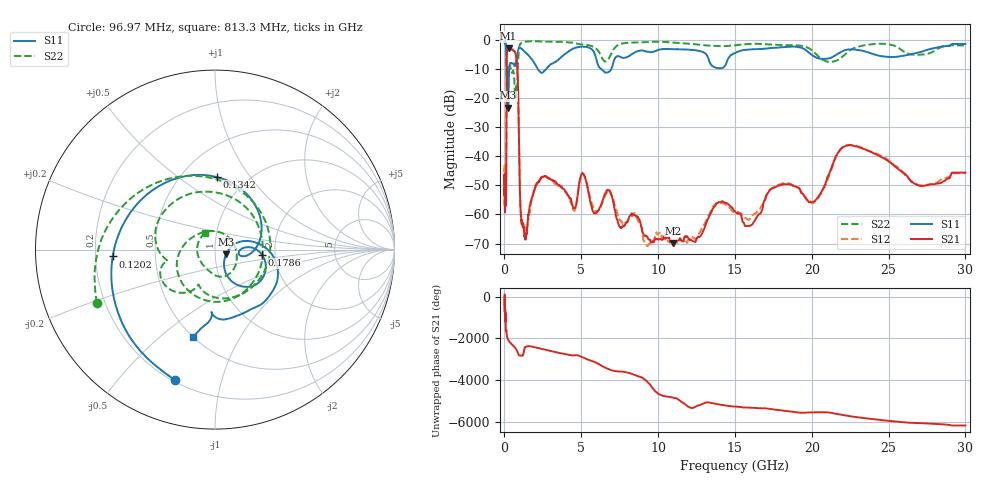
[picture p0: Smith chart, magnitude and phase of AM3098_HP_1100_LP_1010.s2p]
! Date/Time: Thu, Feb 28, 2019 8:44 AM
! Network Analyzer: Agilent Technologies E8364B Rev: A.07.50.67
! Sweep from 0.010 to 30.000 GHz, 1601 Points, Sweep Type: LOG
! Power Supply: 5.023 V, 0.002 A
# Hz S DB R 50
!freq MagS11 AngS11 MagS21 AngS21 MagS12 AngS12 MagS22 AngS22
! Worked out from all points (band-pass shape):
!   1601 points, 10 MHz to 30 GHz, reference 50 ohm
!   highest |S21| = -3.06 dB at 266.5 MHz (marker M1); lowest = -69.8 dB at 10.97 GHz (marker M2)
!   |S21| within 3 dB of the highest: 149.3 MHz to 771.3 MHz (622 MHz wide, 135 % of centre)
!   lowest |S11| = -23.4 dB at 248.4 MHz (marker M3), VSWR 1.15, Z = 56.6 - j2.94 ohm
!   |S11| at or under -10 dB: 140.1 MHz to 314 MHz (173.9 MHz wide, 76.6 % of centre); 2.155 GHz to 2.737 GHz (582.1 MHz wide, 23.8 % of centre); 6.27 GHz to 6.964 GHz (693.1 MHz wide, 10.5 % of centre)
!   |S22| runs from -20.0 to -0.6 dB; largest |S21 - S12| = 0.011
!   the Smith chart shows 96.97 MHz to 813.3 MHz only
!   S11 on the Smith chart (normalised r, x): 96.97 MHz: 0.21, -0.72; 120.2 MHz: 0.27, -0.03; 134.2 MHz: 0.73, +0.71; 178.6 MHz: 1.71, -0.11; 813.3 MHz: 0.50, -0.65
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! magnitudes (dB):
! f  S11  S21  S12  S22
! 10 MHz  -0.3  -46.6  -45.4  -0.6
! 38.04 MHz  -0.4  -55.8  -57.4  -0.8
! 48.61 MHz  -0.6  -46.6  -49.0  -1.1
! 96.97 MHz  -2.4  -55.6  -54.7  -2.8
! 120.2 MHz  -4.9  -37.5  -36.6  -6.3
! 134.2 MHz  -7.9  -15.4  -15.4  -10.2
! 144.7 MHz  -12.2  -7.4  -7.4  -11.7
! 178.6 MHz  -11.6  -4.0  -3.9  -10.2
! 248.4 MHz  -23.4  -3.1  -3.1  -11.3
! 266.5 MHz  -17.8  -3.1  -3.0  -11.1
! 550.5 MHz  -8.1  -3.7  -3.7  -10.7
! 813.3 MHz  -5.9  -8.0  -8.0  -19.3
! 1.098 GHz  -3.1  -61.9  -62.7  -1.2
! 1.389 GHz  -4.5  -68.2  -65.0  -0.7
! 2.084 GHz  -9.3  -49.8  -49.4  -0.6
! 4.503 GHz  -3.1  -57.8  -58.6  -1.1
! 5.128 GHz  -2.4  -46.0  -46.0  -1.7
! 7.926 GHz  -6.1  -62.6  -63.0  -1.2
! 10.97 GHz  -3.3  -69.8  -70.3  -1.1
! 20.1 GHz  -5.6  -55.7  -56.0  -4.1
! 22.56 GHz  -3.4  -36.3  -36.2  -3.5
! 30 GHz  -1.5  -45.7  -45.9  -2.0
